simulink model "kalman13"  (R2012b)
settings: Solver=ode45  StartTime=0.0  StopTime=100  RelTol=1e-3
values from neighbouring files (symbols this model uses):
  dt = 0.01    [aktiv_tilger_1.m]    (also in aktiv_tilger_12.m; aktiv_tilger_2.m; beobachter_1.m; beobachter_2.m)
  Kest = kalman(P,1,0.01),    [LQG_1.m]    (also in ss_zwei_eing_1.m = kalman(sys2, Q, R))
  ki = -Kn(n+1)    [beobachter_2.m]    (also in beobachter_22.m; kalman_12.m = -Kn(3); kalman_13.m = -Kn(4); kalman_d1.m = -Kn(4))
  Kr = 2000    [aktiv_tilger_2.m]    (also in beobachter_22.m = 5; fuellstnd_3.m = 10,; fuellstnd_31.m = 10,; kalman_12.m = Kn(1:2))
  sys2 = sys1(:,[1,1,1])    [kalman_11.m]    (also in kalman_12.m; kalman_13.m = sys1(:,[1,1,1,1]); kalman_2.m = ss(H2); kalman_3.m = ss(H2))
  vnd = 1e-4    (= 0.0001)    [kalman_1.m]    (also in kalman_10.m; kalman_11.m; kalman_12.m; kalman_13.m = 0.01)
  vny = 1e-6    (= 1e-06)    [kalman_1.m]    (also in kalman_10.m; kalman_11.m = ', num2str(vny),' )']); kalman_12.m = ', num2str(vny),' )']); kalman_13.m = ', num2str(vny),' )']))
  x0 = [30,-20,0,0,0,0]    [beobachter_1.m]    (also in beobachter_2.m = [0,0,0,0,0.3,0]; beobachter_22.m = [0.1,0,0.1,0,0.3,0]; kalman_13.m = zeros(1,3); kalman_d1.m = zeros(1,3))
libraries: simulink x2

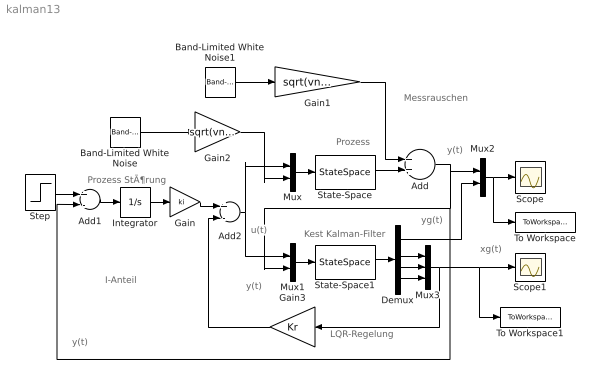
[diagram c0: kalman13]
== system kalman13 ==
  note: I-Anteil
  note: LQR-Regelung
  note: y(t)
  note: y(t)
  note: xg(t)
  note: u(t)
  note: y(t)
  note: yg(t)
  note: Messrauschen
  note: Prozess StÃ¶rung
  note: Kest Kalman-Filter
  note: Prozess
  Add : Sum
  Add1 : Sum  Inputs=+-
  Add2 : Sum  Inputs=+-
  Band-Limited White Noise : simulink/Sources/Band-Limited White Noise  Cov=[dt, dt, dt]  Ts=dt  seed=[23341, 2785, 3672]
  Band-Limited White Noise1 : simulink/Sources/Band-Limited White Noise  Cov=dt  Ts=dt  seed=[23341]
  Demux : Demux
  Gain : Gain  Gain=ki
  Gain1 : Gain  Gain=sqrt(vny)
  Gain2 : Gain  Gain=sqrt(vnd)*eye(3,3)  Multiplication=Matrix(K*u)
  Gain3 : Gain  Gain=Kr  Multiplication=Matrix(K*u)
  Integrator : Integrator
  Mux : Mux  Inputs=2
  Mux1 : Mux  Inputs=2
  Mux2 : Mux  Inputs=2
  Mux3 : Mux  Inputs=3
  Scope : Scope
  Scope1 : Scope
  State-Space : StateSpace  A=sys2.a  B=sys2.b  C=sys2.c  D=sys2.d  X0=x0
  State-Space1 : StateSpace  A=Kest.a  B=Kest.b  C=Kest.c  D=Kest.d
  Step : Step  After=step  SampleTime=0
  To Workspace : ToWorkspace  VariableName=y  SampleTime=-1  SaveFormat=Structure With Time
  To Workspace1 : ToWorkspace  VariableName=y1  SampleTime=-1  SaveFormat=Structure With Time
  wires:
  Mux/1 -> State-Space/1
  Band-Limited White Noise/1 -> Gain2/1
  Gain2/1 -> Mux/2
  Band-Limited White Noise1/1 -> Gain1/1
  State-Space/1 -> Add/2
  Gain1/1 -> Add/1
  Add/1 -> Add1/2, Mux1/2, Mux2/1
  Mux1/1 -> State-Space1/1
  State-Space1/1 -> Demux/1
  Mux2/1 -> To Workspace/1, Scope/1
  Demux/1 -> Mux2/2
  Demux/2 -> Mux3/1
  Demux/3 -> Mux3/2
  Mux3/1 -> Gain3/1, To Workspace1/1, Scope1/1
  Step/1 -> Add1/1
  Add1/1 -> Integrator/1
  Integrator/1 -> Gain/1
  Gain/1 -> Add2/1
  Add2/1 -> Mux1/1, Mux/1
  Gain3/1 -> Add2/2
  Demux/4 -> Mux3/3
